FUNCTION_BLOCK T_SmartLight
VAR
	light : DUT_BalluffSmartLight;
END_VAR

METHOD PUBLIC SwitchAllLampsOff
VAR_INPUT
END_VAR
light.Out.MDP5001_6220_Segment_1_color_IECCONF_IECCONF_Background_color_IECCONF_IECCONF_LED3_1_Bit0 := false;
END_METHOD

END_FUNCTION_BLOCK
